[IBIS VER]   5.0
[File Name]   f28p551rsh.ibs
[File Rev]   1.0
[Date]   August 04, 2025
[Source]   File originated at Texas Instruments
[Copyright]   (c) 2012, Texas Instruments Inc.
[Component]   f28p551rsh
[Manufacturer]  Texas Instruments
[Package]
| Variable   Typ   Min   Max
R_pkg  1.78E-01  8.06E-02  2.46E-01
L_pkg  5.38E-09  4.07E-09  6.46E-09
C_pkg  9.41E-15  6.94E-15   1.85E-14
[Pin]   signal_name   model_name   R_pin   L_pin   C_pin
   1   GPIO6   BCF3385DSHYPBFZ_LC_USF  1.89E-01  5.93E-09  1.76E-14
   2   GPIO29   BCF3385DSHYPBFZ_LC  1.53E-01  5.40E-09  8.24E-15
   3   A16,B16,C16,GPIO28   BCF3385DSHYPBFZ_LC  1.44E-01  5.15E-09  7.88E-15
   4   XRSn   BQ0491FS_USF  1.43E-01  5.00E-09  7.60E-15
   5   VDD   NC  8.68E-02  4.26E-09  8.48E-15
   6   A3,B3,C5,GPIO242,PGA2_INP   BCF3385DSHYPBFZ_LC_USF  1.50E-01  4.76E-09  8.61E-15
   7   A2,B6,C9,GPIO224,PGA1_INP   BCF3385DSHYPBFZ_LC  1.41E-01  4.52E-09  8.19E-15
   8   A15,B9,C7,PGA1_INM   ICF33SHYPB_LC  1.44E-01  4.54E-09  8.21E-15
   9   A14,B14,C4,PGA1_OUT   ICF33SHYPB_LC  1.43E-01  4.69E-09  8.56E-15
   10   A11,B10,C0,PGA2_OUT   ICF33SHYPB_LC  1.41E-01  4.82E-09  8.90E-15
   11   A5,B12,C2,PGA2_INM   ICF33SHYPB_LC  1.49E-01  5.06E-09  7.64E-15
   12   A1,B7,D11,DACB_OUT   ICF33SHYPB_LC  1.68E-01  5.40E-09  8.05E-15
   13   A0,B15,C15,DACA_OUT   ICF33SHYPB_LC  1.92E-01  5.81E-09  8.54E-15
   14   D20,E20,VREFHI   ICF33SHYPB_LC  8.94E-02  4.90E-09  8.04E-15
   15   A13,B13,C13,D13,E13,VREFLO   ICF33SHYPB_LC  8.99E-02  4.94E-09  8.11E-15
   16   A12,C1,E11,PGA3_INP   ICF33SHYPB_LC  2.10E-01  6.03E-09  8.74E-15
   17   A7,B30,C3,D12,E30,PGA3_INM   ICF33SHYPB_LC  2.03E-01  5.80E-09  8.40E-15
   18   A8,B0,C11,PGA3_OUT   ICF33SHYPB_LC  1.99E-01  5.60E-09  8.08E-15
   19   VSSA   NC  8.58E-02  4.28E-09  6.94E-15
   20   VDDA   NC  8.06E-02  4.07E-09  8.15E-15
   21   A4,B8,C14   ICF33SHYPB_LC  1.99E-01  5.14E-09  8.69E-15
   22   A9,B4,C8,GPIO227,GPIO236   BCF3385DSHYPBFZ_LC  1.95E-01  5.10E-09  8.67E-15
   23   A10,B1,C10,GPIO230   BCF3385DSHYPBFZ_LC  1.98E-01  5.29E-09  9.05E-15
   24   A17,B17,C17,CMP1_DACL,GPIO20   BCF3385DSHYPBFZ_LC  2.02E-01  5.48E-09  7.82E-15
   25   A18,B18,C18,GPIO21   BCF3385DSHYPBFZ_LC  1.98E-01  5.60E-09  8.08E-15
   26   A19,B19,C19,GPIO13   BCF3385DSHYPBFZ_LC  2.02E-01  5.79E-09  8.40E-15
   27   A20,B20,C20,GPIO12   BCF3385DSHYPBFZ_LC  2.14E-01  6.07E-09  8.77E-15
   28   A24,D0,E0,GPIO11   BCF3385DSHYPBFZ_LC  2.27E-01  6.35E-09  1.83E-14
   29   B24,D1,E1,GPIO33   BCF3385DSHYPBFZ_LC  2.26E-01  6.31E-09  1.82E-14
   30   C24,D2,E2,GPIO16   BCF3385DSHYPBFZ_LC  2.05E-01  5.94E-09  8.63E-15
   31   A25,D3,E3,GPIO17   BCF3385DSHYPBFZ_LC  1.89E-01  5.62E-09  8.23E-15
   32   B25,D4,E4,GPIO24   BCF3385DSHYPBFZ_LC  1.82E-01  5.39E-09  7.89E-15
   33   TCK   BCF3355DSHYPBFZ_TMS_USF  1.83E-01  5.25E-09  9.22E-15
   34   GPIO37/TDO   BCPF335585DSHYPBFZ  1.79E-01  5.06E-09  8.83E-15
   35   TMS   BCF3355DSHYPBFZ_TMS  1.83E-01  4.94E-09  8.50E-15
   36   GPIO35/TDI   BCF3385DSHYPBFZ_LC  1.95E-01  5.07E-09  8.59E-15
   37   GPIO32   BQ3320HYPBFZ_3VSBLK_5FS_LC  2.09E-01  5.37E-09  9.06E-15
   38   GPIO18,X2   BCF3385DSHYPBFZ_LC  1.94E-01  5.37E-09  9.30E-15
   39   GPIO19,X1   BCPF335585DSHYPBFZ  2.07E-01  5.65E-09  8.08E-15
   40   VDDIO   NC  2.23E-01  5.97E-09  8.49E-15
   41   VDD   NC  1.28E-01  5.14E-09  8.05E-15
   42   VREGENZ   IQ0440FS_VREGENZ_USF  2.27E-01  6.32E-09  1.82E-14
   43   GPIO4   BCF3385DSHYPBFZ_LC  2.09E-01  6.17E-09  1.80E-14
   44   GPIO3  BQ3320HYPBFZ_3VSBLK_5FS_LC  1.84E-01  5.76E-09  8.54E-15
   45   GPIO2  BQ3320HYPBFZ_3VSBLK_5FS_LC  1.77E-01  5.54E-09  8.21E-15
   46   GPIO1   BCF3385DSHYPBFZ_LC  1.70E-01  5.31E-09  7.87E-15
   47   GPIO0   BCF3385DSHYPBFZ_LC  1.68E-01  5.13E-09  7.56E-15
   48   GPIO40   BCF3385DSHYPBFZ_LC  1.75E-01  5.04E-09  8.87E-15
   49   GPIO23   BCF3385DSHYPBFZ_LC  1.83E-01  4.98E-09  8.58E-15
   50   GPIO41   BCF3385DSHYPBFZ_LC  1.99E-01  5.14E-09  8.70E-15
   51   GPIO22   BCF3385DSHYPBFZ_LC  2.15E-01  5.46E-09  9.18E-15
   52   GPIO7   BCF3385DSHYPBFZ_LC  2.42E-01  5.90E-09  8.13E-15
   53   VDD   NC  1.20E-01  4.79E-09  7.48E-15
   54   VDDIO   NC  2.33E-01  6.10E-09  8.62E-15
   55   GPIO5   BCF3385DSHYPBFZ_LC  2.13E-01  6.05E-09  8.76E-15
   56   GPIO9  BQ3320HYPBFZ_3VSBLK_5FS_LC  2.38E-01  6.46E-09  1.85E-14
| End of package information
|   Component BQ0491FS_USF
[Component]   BQ0491FS_USF
[Manufacturer]   Texas Instruments
[Package]
|  variable   typ   min   max
R_pkg   0   0   0
L_pkg   0   0   0
C_pkg   0   0   0
[Pin]   signal_name   model_name   R_pin   L_pin   C_pin
VSS   VSS   GND
VDDS   VDDS   POWER
PAD   PAD   BQ0491FS_USF
[Model Selector] BQ0491FS_USF
WK_PU_ON_WITH_RX_3P3  Cell operated at 3.3(nom)
|WK_PU_ON_WITH_RX_3P3; WEAK_PULLUP_ON_WITH_RX
OPEN_DRAIN_MODE_3P3  Cell operated at 3.3(nom)
|   Component BCPF335585DSHYPBFZ
[Component]   BCPF335585DSHYPBFZ
[Manufacturer]   Texas Instruments
[Package]
|  variable   typ   min   max
R_pkg   0   0   0
L_pkg   0   0   0
C_pkg   0   0   0
[Pin]   signal_name   model_name   R_pin   L_pin   C_pin
VSS   VSS   GND
VDDS   VDDS   POWER
PAD   PAD   BCPF335585DSHYPBFZ
[Model Selector] BCPF335585DSHYPBFZ
BCPF_WK_PU_ON_3P3  Cell operated at 3.3(nom)
|BCPF_WK_PU_ON_3P3; WEAK_PULLUP_ON
BCPF_DRIVER_MODE_4MA_3P3  Cell operated at 3.3(nom)
|BCPF_DRIVER_MODE_4MA_3P3
BCPF_DRIVER_MODE_2MA_3P3  Cell operated at 3.3(nom)
|BCPF_DRIVER_MODE_2MA_3P3
BCPF_WK_PD_ON_3P3  Cell operated at 3.3(nom)
|   Component ICF33SHYPB_LC
[Component]   ICF33SHYPB_LC
[Manufacturer]   Texas Instruments
[Package]
|  variable   typ   min   max
R_pkg   0   0   0
L_pkg   0   0   0
C_pkg   0   0   0
[Pin]   signal_name   model_name   R_pin   L_pin   C_pin
VSS   VSS   GND
VDDS   VDDS   POWER
PAD   PAD   ICF33SHYPB_LC
[Model Selector] ICF33SHYPB_LC
ICF_RECEIVER_MODE_3P3  Cell operated at 3.3(nom)
|ICF_RECEIVER_MODE_3P3; RECEIVER_MODE
ICF_WK_PU_ON_3P3  Cell operated at 3.3(nom)
|ICF_WK_PU_ON_3P3; WEAK_PULLUP_ON
ICF_WK_PD_ON_3P3  Cell operated at 3.3(nom)
|   Component BCF3385DSHYPBFZ_LC_USF
[Component]   BCF3385DSHYPBFZ_LC_USF
[Manufacturer]   Texas Instruments
[Package]
|  variable   typ   min   max
R_pkg   0   0   0
L_pkg   0   0   0
C_pkg   0   0   0
[Pin]   signal_name   model_name   R_pin   L_pin   C_pin
VSS   VSS   GND
VDDS   VDDS   POWER
PAD   PAD   BCF3385DSHYPBFZ_LC_USF
[Model Selector] BCF3385DSHYPBFZ_LC_USF
BCF_WK_PU_ON_3P3  Cell operated at 3.3(nom)
|BCF_WK_PU_ON_3P3; WEAK_PULLUP_ON
BCF_WK_PD_ON_3P3  Cell operated at 3.3(nom)
|BCF_WK_PD_ON_3P3; WEAK_PULLDOWN_ON
BCF_DRIVER_MODE_3P3  Cell operated at 3.3(nom)
|BCF_DRIVER_MODE_3P3
BCF_RECEIVER_MODE_3P3  Cell operated at 3.3(nom)
|   Component BCF3355DSHYPBFZ_TMS_USF
[Component]   BCF3355DSHYPBFZ_TMS_USF
[Manufacturer]   Texas Instruments
[Package]
|  variable   typ   min   max
R_pkg   0   0   0
L_pkg   0   0   0
C_pkg   0   0   0
[Pin]   signal_name   model_name   R_pin   L_pin   C_pin
VSS   VSS   GND
VDDS   VDDS   POWER
PAD   PAD   BCF3355DSHYPBFZ_TMS_USF
[Model Selector] BCF3355DSHYPBFZ_TMS_USF
TMS_WK_PU_ON_3P3  Cell operated at 3.3(nom)
|TMS_WK_PU_ON_3P3; WEAK_PULLUP_ON
TMS_DRIVER_3P3  Cell operated at 3.3(nom)
|TMS_DRIVER_3P3
TMS_WK_PD_ON_3P3  Cell operated at 3.3(nom)
|   Component BCF3385DSHYPBFZ_LC
[Component]   BCF3385DSHYPBFZ_LC
[Manufacturer]   Texas Instruments
[Package]
|  variable   typ   min   max
R_pkg   0   0   0
L_pkg   0   0   0
C_pkg   0   0   0
[Pin]   signal_name   model_name   R_pin   L_pin   C_pin
VSS   VSS   GND
VDDS   VDDS   POWER
PAD   PAD   BCF3385DSHYPBFZ_LC
[Model Selector] BCF3385DSHYPBFZ_LC
BCF_WK_PU_ON_3P3  Cell operated at 3.3(nom)
|BCF_WK_PU_ON_3P3; WEAK_PULLUP_ON
BCF_WK_PD_ON_3P3  Cell operated at 3.3(nom)
|BCF_WK_PD_ON_3P3; WEAK_PULLDOWN_ON
BCF_DRIVER_MODE_3P3  Cell operated at 3.3(nom)
|BCF_DRIVER_MODE_3P3
BCF_RECEIVER_MODE_3P3  Cell operated at 3.3(nom)
|BCF_RECEIVER_MODE_3P3; RECEIVER_MODE
|   Component IQ0440FS_VREGENZ_USF
[Component]   IQ0440FS_VREGENZ_USF
[Manufacturer]   Texas Instruments
[Package]
|  variable   typ   min   max
R_pkg   0   0   0
L_pkg   0   0   0
C_pkg   0   0   0
[Pin]   signal_name   model_name   R_pin   L_pin   C_pin
VSS   VSS   GND
VDDS   VDDS   POWER
PAD   PAD   IQ0440FS_VREGENZ_USF
[Model Selector] IQ0440FS_VREGENZ_USF
VREGENZ_WK_PD_ON_3P3  Cell operated at 3.3(nom)
|VREGENZ_WK_PD_ON_3P3; WEAK_PULLDOWN_ON
VREGENZ_WK_PD_OFF_3P3  Cell operated at 3.3(nom)
|   Component BCF3355DSHYPBFZ_TMS
[Component]   BCF3355DSHYPBFZ_TMS
[Manufacturer]   Texas Instruments
[Package]
|  variable   typ   min   max
R_pkg   0   0   0
L_pkg   0   0   0
C_pkg   0   0   0
[Pin]   signal_name   model_name   R_pin   L_pin   C_pin
VSS   VSS   GND
VDDS   VDDS   POWER
PAD   PAD   BCF3355DSHYPBFZ_TMS
[Model Selector] BCF3355DSHYPBFZ_TMS
TMS_WK_PU_ON_3P3  Cell operated at 3.3(nom)
|TMS_WK_PU_ON_3P3; WEAK_PULLUP_ON
TMS_DRIVER_3P3  Cell operated at 3.3(nom)
|TMS_DRIVER_3P3
TMS_WK_PD_ON_3P3  Cell operated at 3.3(nom)
|TMS_WK_PD_ON_3P3; WEAK_PULLDOWN_ON
|   Component BQ3320HYPBFZ_3VSBLK_5FS_LC
[Component] BQ3320HYPBFZ_3VSBLK_5FS_LC
[Manufacturer] Texas Instruments
[Package]
| variable   typ   min   max
R_pkg   0.0   0.0   0.0
L_pkg   0.0H   0.0H   0.0H
C_pkg   0.0F   0.0F   0.0F
[Pin]  signal_name   model_name   R_pin   L_pin   C_pin
PAD   PAD   BQ3320HYPBFZ_3VSBLK_5FS_LC
VDDS   VDDS   Power
VSS   VSS   Gnd
A   A   NC
GZ   GZ   NC
[Model Selector] BQ3320HYPBFZ_3VSBLK_5FS_LC
BQ3320HYPBFZ_3VSBLK_5FS_LC_M0_D0 I/O model with Mode = 0 and Drive = 0
BQ3320HYPBFZ_3VSBLK_5FS_LC_M0_D1 I/O model with Mode = 0 and Drive = 1
BQ3320HYPBFZ_3VSBLK_5FS_LC_M1_D0 I/O model with Mode = 1 and Drive = 0
BQ3320HYPBFZ_3VSBLK_5FS_LC_M1_D1 I/O model with Mode = 1 and Drive = 1
BQ3320HYPBFZ_3VSBLK_5FS_LC_PDON I/O model with Pulldown on PI=0 PSEL=0
BQ3320HYPBFZ_3VSBLK_5FS_LC_PUON I/O model with Pullup on PI=0 PSEL=0
| Models and submodels in the file (24): WK_PU_ON_WITH_RX_3P3 (Input), OPEN_DRAIN_MODE_3P3 (I/O_open_drain), BCPF_WK_PU_ON_3P3 (Input), BCPF_DRIVER_MODE_4MA_3P3 (I/O), BCPF_DRIVER_MODE_2MA_3P3 (I/O), BCPF_WK_PD_ON_3P3 (Input), ICF_RECEIVER_MODE_3P3 (Input), ICF_WK_PU_ON_3P3 (Input), ICF_WK_PD_ON_3P3 (Input), BCF_WK_PU_ON_3P3 (Input), BCF_WK_PD_ON_3P3 (Input), BCF_DRIVER_MODE_3P3 (I/O), BCF_RECEIVER_MODE_3P3 (Input), TMS_WK_PU_ON_3P3 (Input), TMS_DRIVER_3P3 (I/O), TMS_WK_PD_ON_3P3 (Input), VREGENZ_WK_PD_ON_3P3 (Input), VREGENZ_WK_PD_OFF_3P3 (Input), BQ3320HYPBFZ_3VSBLK_5FS_LC_M0_D0 (I/O), BQ3320HYPBFZ_3VSBLK_5FS_LC_M0_D1 (I/O), BQ3320HYPBFZ_3VSBLK_5FS_LC_M1_D0 (I/O), BQ3320HYPBFZ_3VSBLK_5FS_LC_M1_D1 (I/O), BQ3320HYPBFZ_3VSBLK_5FS_LC_PDON (Input), BQ3320HYPBFZ_3VSBLK_5FS_LC_PUON (Input)
